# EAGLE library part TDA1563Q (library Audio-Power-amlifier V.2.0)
The TDA1563Q is a monolithic power amplifier in a 17-lead DIL-bent-SIL plastic power package. It contains two identical 25 Wamplifiers. The dissipation is minimized by switching from SE to BTL mode when a higher output voltage swing is needed. The device is primarily developed for car radio applications.
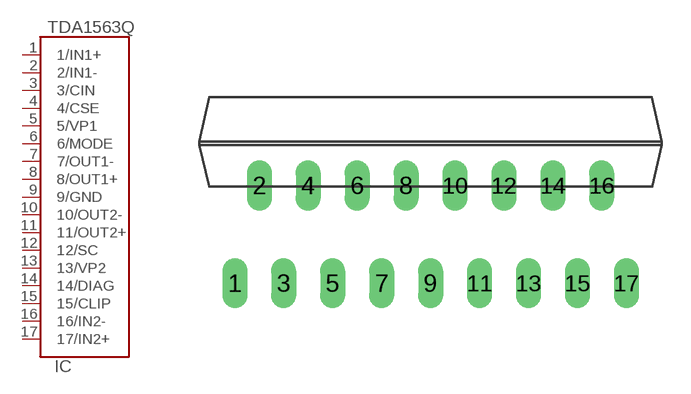
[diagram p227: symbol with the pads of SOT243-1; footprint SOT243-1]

Designator prefix IC

## TDA1563Q  [SOT243-1]
1  1/IN1+  in
2  2/IN1-  in
3  3/CIN  in
4  4/CSE
5  5/VP1  pwr
6  6/MODE  in
7  7/OUT1-  out
8  8/OUT1+  out
9  9/GND  pwr
10  10/OUT2-  out
11  11/OUT2+  out
12  12/SC
13  13/VP2  pwr
14  14/DIAG
15  15/CLIP
16  16/IN2-  in
17  17/IN2+  in

## Footprint SOT243-1 (pad centres in mm)
DBS17P: plastic DIL-bent-SIL power package; 17 leads (lead length 7.7 mm)
drill 0.8 long: 1 -10.16,-5.08; 2 -8.89,0; 3 -7.62,-5.08; 4 -6.35,0; 5 -5.08,-5.08; 6 -3.81,0; 7 -2.54,-5.08; 8 -1.27,0; 9 0,-5.08; 10 1.27,0; 11 2.54,-5.08; 12 3.81,0; 13 5.08,-5.08; 14 6.35,0; 15 7.62,-5.08; 16 8.89,0; 17 10.17,-5.08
